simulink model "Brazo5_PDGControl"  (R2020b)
settings: Solver=VariableStepAuto  StartTime=0.0  StopTime=10.0  RelTol=1e-3
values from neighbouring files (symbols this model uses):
  b = 0.02    [robotSimulationWithConstraints.m]
  J = 0.01    [robotSimulationWithConstraints.m]
  K = 0.75    [robotSimulationWithConstraints.m]
  L = 1.1*10^-3    (= 0.0011)    [robotSimulationWithConstraints.m]
  qd = q    [robotSimulationWithConstraints.m]
  R = 5.2    [robotSimulationWithConstraints.m]
undefined symbols (not defined in the file or in its folder): deg, kg, m, N, rad, s, X, Y, Z
libraries: sm_lib x59, nesl_utility x16, robotmaniplib x1
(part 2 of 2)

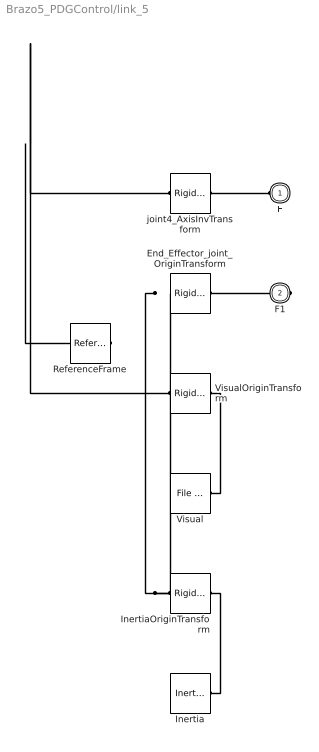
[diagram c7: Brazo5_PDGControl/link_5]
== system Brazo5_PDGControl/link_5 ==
  End_Effector_joint_OriginTransform : sm_lib/Frames and Transforms/Rigid Transform  TranslationMethod=Cartesian  TranslationStandardOffset=0  TranslationLengthUnit=m  TranslationStandardAxis=+Z  TranslationCartesianOffset=[0, 0, 0.1005]  TranslationROffset=0  TranslationROffsetUnits=m  TranslationZOffset=0  TranslationZOffsetUnits=m  TranslationThetaOffset=0  TranslationThetaOffsetUnits=deg  RotationMethod=RotationSequence  RotationAngleUnits=deg  RotationStandardAxis=+Z  RotationAngle=0.0  RotationArbitraryAxis=[0 0 1]  FollAlignAxisA=+X  BaseAlignAxisA=+Y  FollAlignAxisB=+Y  BaseAlignAxisB=+Z  RotationSequenceAxes=BaseAxes  RotationSequence=XYZ  RotationSequenceAngles=[0, 0, 0.045381]  RotationSequenceAnglesUnits=rad  RotationMatrix=[1 0 0; 0 1 0; 0 0 1]
  Inertia : sm_lib/Body Elements/Inertia  InertiaType=Custom  Mass=1.4886  MassUnits=kg  CenterOfMass=[0, 0, 0]  CenterOfMassUnits=m  MomentsOfInertia=[0.00086527, 0.00086527, 0.0015073]  MomentsOfInertiaUnits=kg*m^2  ProductsOfInertia=[-1.5349e-20, -1.2683e-19, -7.4327e-21]  ProductsOfInertiaUnits=kg*m^2  GraphicType=None  MarkerShape=Inertia  MarkerSize=20  GraphicVisPropType=SimpleVisualProperties  GraphicDiffuseColor=[0.5 0.5 0.5]  GraphicSpecularColor=[0.5 0.5 0.5 1.0]  GraphicAmbientColor=[0.15 0.15 0.15 1.0]  GraphicEmissiveColor=[0.0 0.0 0.0 1.0]  GraphicShininess=75  GraphicOpacity=1.0
  InertiaOriginTransform : sm_lib/Frames and Transforms/Rigid Transform  TranslationMethod=Cartesian  TranslationStandardOffset=0  TranslationLengthUnit=m  TranslationStandardAxis=+Z  TranslationCartesianOffset=[1.1102e-16, -1.5173e-17, 0.08550000000000001]  TranslationROffset=0  TranslationROffsetUnits=m  TranslationZOffset=0  TranslationZOffsetUnits=m  TranslationThetaOffset=0  TranslationThetaOffsetUnits=deg  RotationMethod=RotationSequence  RotationAngleUnits=deg  RotationStandardAxis=+Z  RotationAngle=0.0  RotationArbitraryAxis=[0 0 1]  FollAlignAxisA=+X  BaseAlignAxisA=+Y  FollAlignAxisB=+Y  BaseAlignAxisB=+Z  RotationSequenceAxes=BaseAxes  RotationSequence=XYZ  RotationSequenceAngles=[0, 0, 0]  RotationSequenceAnglesUnits=rad  RotationMatrix=[1 0 0; 0 1 0; 0 0 1]
  ReferenceFrame : sm_lib/Frames and Transforms/Reference Frame
  Visual : sm_lib/Body Elements/File Solid  ExtGeomFileName=Brazo5_SLDASM/meshes/link_5.STL  UnitType=Custom  ExtGeomFileUnits=m  StepReaderType=HEX  ExportConvexHullGeometry=off  InertiaType=Custom  Mass=0  MassUnits=kg  CenterOfMass=[0, 0, 0]  CenterOfMassUnits=m  MomentsOfInertia=[0, 0, 0]  MomentsOfInertiaUnits=kg*m^2  ProductsOfInertia=[0, 0, 0]  ProductsOfInertiaUnits=kg*m^2  BasedOnType=DensityFromFile  Density=1000  DensityUnits=kg/m^3  DoExposeReferenceFrame=on  SerializedFrames=<Frames/>  GraphicType=FromGeometry  MarkerShape=Sphere  MarkerSize=10  GraphicVisPropType=SimpleVisualProperties  GraphicDiffuseColor=[0.77647, 0.75686, 0.73725]  GraphicSpecularColor=[0.5 0.5 0.5 1.0]  GraphicAmbientColor=[0.15 0.15 0.15 1.0]  GraphicEmissiveColor=[0.0 0.0 0.0 1.0]  GraphicShininess=75  GraphicOpacity=1
  VisualOriginTransform : sm_lib/Frames and Transforms/Rigid Transform  TranslationMethod=Cartesian  TranslationStandardOffset=0  TranslationLengthUnit=m  TranslationStandardAxis=+Z  TranslationCartesianOffset=[0, 0, 0]  TranslationROffset=0  TranslationROffsetUnits=m  TranslationZOffset=0  TranslationZOffsetUnits=m  TranslationThetaOffset=0  TranslationThetaOffsetUnits=deg  RotationMethod=RotationSequence  RotationAngleUnits=deg  RotationStandardAxis=+Z  RotationAngle=0.0  RotationArbitraryAxis=[0 0 1]  FollAlignAxisA=+X  BaseAlignAxisA=+Y  FollAlignAxisB=+Y  BaseAlignAxisB=+Z  RotationSequenceAxes=BaseAxes  RotationSequence=XYZ  RotationSequenceAngles=[0, 0, 0]  RotationSequenceAnglesUnits=rad  RotationMatrix=[1 0 0; 0 1 0; 0 0 1]
  joint4_AxisInvTransform : sm_lib/Frames and Transforms/Rigid Transform  TranslationMethod=Cartesian  TranslationStandardOffset=0  TranslationLengthUnit=m  TranslationStandardAxis=+Z  TranslationCartesianOffset=[0, 0, 0]  TranslationROffset=0  TranslationROffsetUnits=m  TranslationZOffset=0  TranslationZOffsetUnits=m  TranslationThetaOffset=0  TranslationThetaOffsetUnits=deg  RotationMethod=ArbitraryAxis  RotationAngleUnits=rad  RotationStandardAxis=+Z  RotationAngle=0  RotationArbitraryAxis=[1, 0, 0]  FollAlignAxisA=+X  BaseAlignAxisA=+Y  FollAlignAxisB=+Y  BaseAlignAxisB=+Z  RotationSequenceAxes=FollowerAxes  RotationSequence=XYX  RotationSequenceAngles=[0 0 0]  RotationSequenceAnglesUnits=deg  RotationMatrix=[1 0 0; 0 1 0; 0 0 1]
  F : PMIOPort  Side=Left
  F1 : PMIOPort  Port=2  Side=Right
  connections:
  End_Effector_joint_OriginTransform/RConn1 -- F1/RConn1
  Inertia/RConn1 -- InertiaOriginTransform/RConn1
  InertiaOriginTransform/LConn1 -- End_Effector_joint_OriginTransform/LConn1 -- ReferenceFrame/RConn1 -- VisualOriginTransform/LConn1 -- joint4_AxisInvTransform/LConn1
  Visual/RConn1 -- VisualOriginTransform/RConn1
  joint4_AxisInvTransform/RConn1 -- F/RConn1
